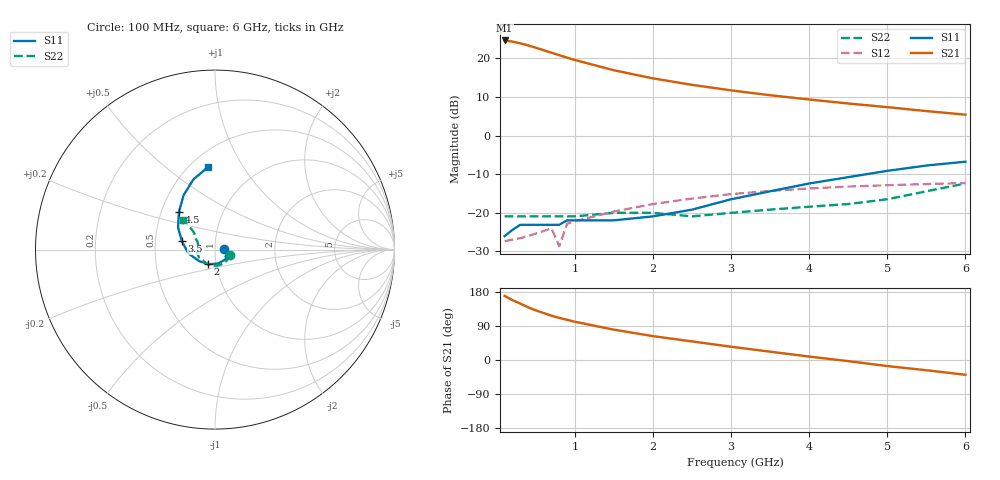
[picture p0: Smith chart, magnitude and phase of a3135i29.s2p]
!  MSA-3135  S AND NOISE PARAMETERS
!  Id = 29 mA LAST UPDATED 06-27-94
# ghz s ma r 50
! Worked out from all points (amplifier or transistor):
!   20 points, 100 MHz to 6 GHz, reference 50 ohm
!   highest |S21| = 24.7 dB at 100 MHz (marker M1)
!   |S21| within 3 dB of that: start of sweep to 672 MHz
!   unconditionally stable (mu >= 1): start of sweep to end of sweep
!   at 400 MHz: K = 1.04, MAG = 23.5 dB, |S12| = -26.0 dB
!   at 1.5 GHz: K = 1.03, MAG = 17.2 dB, |S12| = -19.7 dB
!   at 6 GHz: K = 1.02, MAG = 7.9 dB, |S12| = -12.3 dB
!   S11 on the Smith chart (normalised r, x): 100 MHz: 1.11, +0.00; 2 GHz: 0.91, -0.15; 3.5 GHz: 0.69, +0.07; 4.5 GHz: 0.62, +0.28; 6 GHz: 0.61, +0.71
0.1  0.05 1.0  17.11 169.0  0.043 7.0  0.09 -19.0
0.2  0.06 2.0  16.52 158.0  0.045 14.0  0.09 -37.0
0.3  0.07 -2.0  15.72 149.0  0.047 20.0  0.09 -52.0
0.4  0.07 -7.0  14.77 139.0  0.05 24.0  0.09 -67.0
0.5  0.07 -12.0  13.77 131.0  0.054 29.0  0.09 -80.0
0.6  0.07 -21.0  12.79 124.0  0.058 32.0  0.09 -92.0
0.7  0.07 -27.0  11.86 117.0  0.063 34.0  0.09 -102.0
0.8  0.07 -33.0  11.03 111.0  0.037 36.0  0.09 -111.0
0.9  0.08 -39.0  10.25 106.0  0.072 38.0  0.09 -119.0
1  0.08 -44.0  9.55 101.0  0.078 39.0  0.09 -127.0
1.5  0.08 -79.0  7.03 80.0  0.104 39.0  0.1 -155.0
2  0.09 -116.0  5.52 63.0  0.13 36.0  0.1 -171.0
2.5  0.11 -145.0  4.55 49.0  0.153 31.0  0.09 176.0
3  0.15 -172.0  3.86 35.0  0.175 25.0  0.1 162.0
3.5  0.19 166.0  3.34 22.0  0.192 19.0  0.11 154.0
4  0.24 149.0  2.94 9.0  0.207 13.0  0.12 152.0
4.5  0.29 134.0  2.61 -3.0  0.219 7.0  0.13 148.0
5  0.35 120.0  2.34 -16.0  0.228 1.0  0.15 141.0
5.5  0.41 107.0  2.08 -27.0  0.236 -5.0  0.19 138.0
6  0.46 95.0  1.87 -39.0  0.243 -10.0  0.24 137.0
